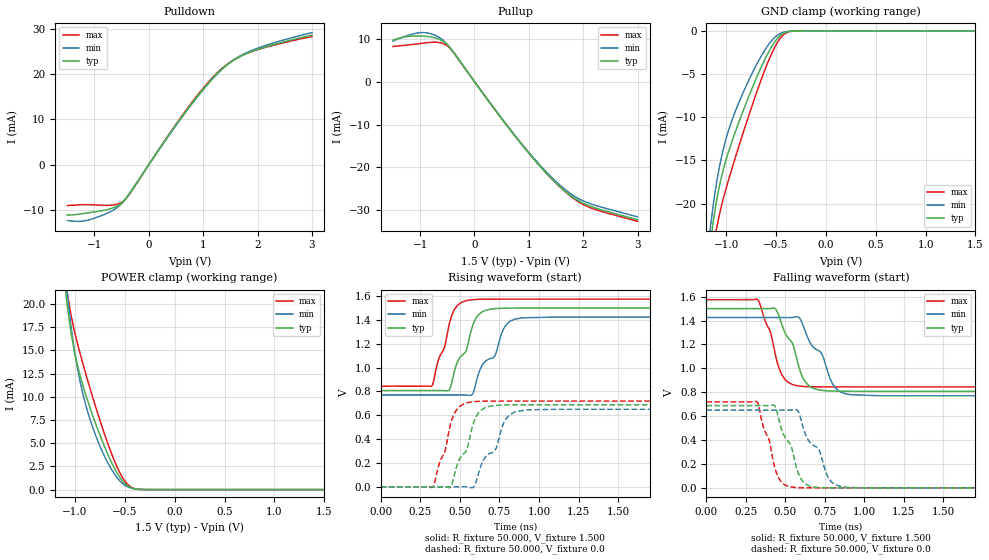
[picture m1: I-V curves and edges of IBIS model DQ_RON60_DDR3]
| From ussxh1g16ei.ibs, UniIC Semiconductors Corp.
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|   Model DQ_RON60_DDR3
[Model] DQ_RON60_DDR3
Model_type I/O
Vinl =  0.615V
Vinh =  0.885V
Vmeas =  0.750V
Rref =  50.000
Vref =  0.750V
C_comp   1.232pF   1.219pF   1.235pF
[Model Spec]
Vinh   0.885V   0.847V   0.922V
Vinl   0.615V   0.577V   0.652V
Vmeas   0.750V   0.712V   0.787V
Vref   0.750V   0.712V   0.787V
Rref   50.000   NA   NA
[Temperature Range]   25.000   95.000   -40.000
[Voltage Range]   1.500V   1.425V   1.575V
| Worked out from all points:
|   slope of the pulldown table from 0 to 0.225 V, typ, clamps not added: 55.6 ohm
|   slope of the pullup table from 0 to 0.225 V, typ, clamps not added: 56.8 ohm
|   GND clamp passes 1 mA (typ) near -0.49 V on its own axis
|   POWER clamp passes 1 mA (typ) near -0.53 V on its own axis
|   rising waveform, R_fixture 50.000, V_fixture 1.500: 20-80 % time 122ps typ, 159ps min, 96.2ps max; typ from 0.808 V to 1.5 V
|   rising waveform, R_fixture 50.000, V_fixture 0.0: 20-80 % time 117ps typ, 151ps min, 93.2ps max; typ from 0 V to 0.688 V
|   falling waveform, R_fixture 50.000, V_fixture 1.500: 20-80 % time 123ps typ, 157ps min, 98.8ps max; typ from 1.5 V to 0.808 V
|   falling waveform, R_fixture 50.000, V_fixture 0.0: 20-80 % time 115ps typ, 148ps min, 90.7ps max; typ from 0.688 V to 0 V
[Pulldown]
|Voltage   I(typ)   I(min)   I(max)
-1.5V     -11.15mA   -12.39mA   -9.054mA
-1.224V   -10.85mA   -12.51mA   -8.863mA
-1.04V    -10.53mA   -12.01mA   -8.882mA
-672mV    -9.631mA   -10.2mA    -8.963mA
-488mV    -8.379mA   -8.453mA   -8.247mA
-350mV    -6.339mA   -6.245mA   -6.423mA
754mV     12.99mA    12.83mA    13.18mA
1.076V    17.8mA     17.67mA    18mA
1.352V    21.22mA    21.19mA    21.38mA
1.582V    23.27mA    23.37mA    23.36mA
1.904V    25.1mA     25.34mA    25.08mA
3V        28.67mA    29.24mA    28.37mA
[Pullup]
|Voltage   I(typ)   I(min)   I(max)
-1.5V     9.689mA    9.449mA    8.196mA
-1.14V    10.61mA    11.09mA    8.66mA
-910mV    10.58mA    11.42mA    9.014mA
-680mV    10.03mA    10.53mA    9.164mA
-496mV    8.577mA    8.63mA     8.309mA
-358mV    6.405mA    6.362mA    6.317mA
746mV     -12.72mA   -12.56mA   -12.64mA
1.16V     -19.08mA   -18.83mA   -19.02mA
1.528V    -23.99mA   -23.63mA   -24.02mA
1.804V    -26.9mA    -26.45mA   -27.06mA
2.034V    -28.56mA   -28mA      -28.86mA
3V        -32.21mA   -31.53mA   -32.56mA
[GND_clamp]
|Voltage   I(typ)   I(min)   I(max)
-1.5V     -77.15mA   -73.99mA   -84.26mA
-1.159V   -24.58mA   -22.75mA   -27.74mA
-1.128V   -21.88mA   -19.96mA   -25.03mA
-1.097V   -19.64mA   -17.59mA   -22.88mA
-1.066V   -17.82mA   -15.61mA   -21.14mA
-1.004V   -15mA      -12.58mA   -18.36mA
-880mV    -10.79mA   -8.48mA    -13.61mA
-632mV    -3.776mA   -2.594mA   -5.119mA
-477mV    -756.2uA   -431.9uA   -1.164mA
-415mV    -225.6uA   -131.2uA   -354.1uA
-322mV    -19.15uA   -14.82uA   -24.1uA
1.5V      0A         0A         0A
[POWER_clamp]
|Voltage   I(typ)   I(min)   I(max)
-1.5V     91.1mA     92.64mA    94.46mA
-1.104V   22.28mA    23.97mA    23.43mA
-1.073V   19.41mA    20.63mA    20.89mA
-1.042V   17.07mA    17.76mA    18.91mA
-980mV    13.62mA    13.3mA     15.93mA
-918mV    11.11mA    10.16mA    13.45mA
-856mV    9.013mA    7.787mA    11.15mA
-670mV    3.78mA     2.864mA    4.931mA
-577mV    1.775mA    1.269mA    2.414mA
-484mV    502.3uA    362.1uA    693.5uA
-329mV    12.96uA    15.92uA    9.805uA
1.5V      0A         0A         0A
[Ramp]
| variable   typ   min   max
dV/dt_r   0.413/0.117n   0.390/0.151n   0.432/93.372p
dV/dt_f   0.415/0.123n   0.393/0.157n   0.438/98.884p
R_load = 50.000
[Rising Waveform]
R_fixture= 50.000
V_fixture= 1.500
V_fixture_min= 1.425
V_fixture_max= 1.575
|time   V(typ)   V(min)   V(max)
0s        808mV      770.4mV    844.7mV
324ps     808.1mV    770.4mV    847.2mV
430ps     808.9mV    770.4mV    1.346V
453ps     898.8mV    770.4mV    1.452V
551ps     1.195V     768.1mV    1.565V
585ps     1.367V     790.6mV    1.571V
623ps     1.45V      969.1mV    1.573V
784ps     1.499V     1.344V     1.575V
848ps     1.5V       1.407V     1.575V
3ns       1.5V       1.425V     1.575V
[Rising Waveform]
R_fixture= 50.000
V_fixture= 0.0
V_fixture_min= 0.0
V_fixture_max= 0.0
|time   V(typ)   V(min)   V(max)
0s        174.5nV    711.1nV    72.81nV
327ps     -9.262uV   8.057uV    -4.838mV
407ps     -269uV     15.12uV    303.3mV
444ps     4.377mV    -14.11uV   538.4mV
563ps     416.1mV    -5.337mV   709.9mV
593ps     560.3mV    10.1mV     714.8mV
636ps     644mV      186.7mV    717.8mV
718ps     681.6mV    295.6mV    719.2mV
850ps     688mV      630mV      719.4mV
3ns       688.4mV    650.7mV    719.4mV
[Falling Waveform]
R_fixture= 50.000
V_fixture= 1.500
V_fixture_min= 1.425
V_fixture_max= 1.575
|time   V(typ)   V(min)   V(max)
0s        1.5V       1.425V     1.575V
324ps     1.5V       1.425V     1.576V
441ps     1.493V     1.425V     1.094V
496ps     1.305V     1.425V     911.4mV
580ps     1.044V     1.432V     853.6mV
657ps     847.6mV    1.216V     846.2mV
730ps     815.9mV    1.125V     845mV
812ps     809.4mV    844.7mV    844.8mV
882ps     808.3mV    787.1mV    844.7mV
3ns       808mV      770.4mV    844.7mV
[Falling Waveform]
R_fixture= 50.000
V_fixture= 0.0
V_fixture_min= 0.0
V_fixture_max= 0.0
|time   V(typ)   V(min)   V(max)
0s        688.4mV    650.7mV    719.4mV
323ps     688.4mV    650.6mV    717.3mV
444ps     653.9mV    650.6mV    125.7mV
536ps     354mV      651.2mV    7.756mV
580ps     132.3mV    645.7mV    2.003mV
628ps     33.83mV    444.5mV    454.2uV
714ps     2.688mV    316.6mV    31.88uV
780ps     383.3uV    70.26mV    4.338uV
864ps     31.35uV    7.026mV    591.4nV
3ns       348.6nV    799nV      264.2nV
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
